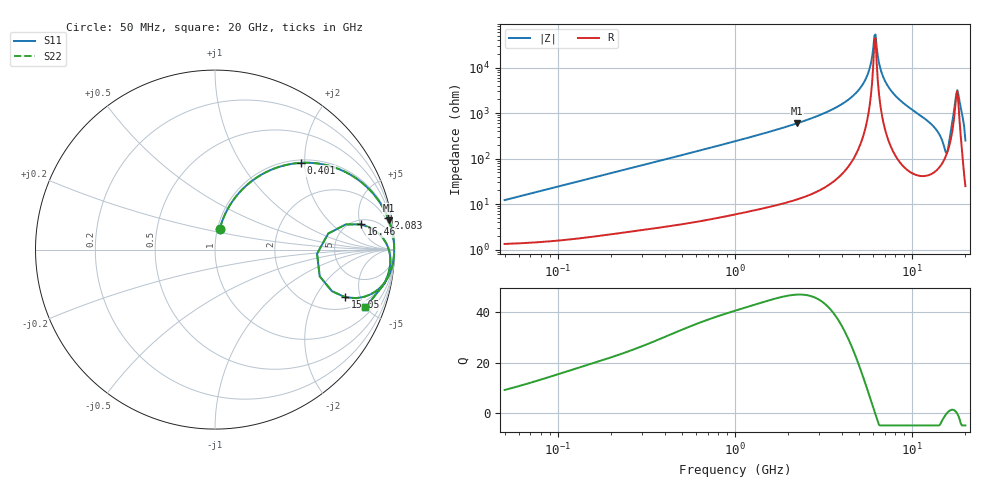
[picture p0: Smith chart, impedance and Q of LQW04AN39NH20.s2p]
!Murata Part Number: LQW04AN39NH20
!These Parameters are Measured in Series Mode Connection
!  o--[Z]--o
!Port1  Port2
!  o-------o
!Freq. Start=50[MHz] Stop=20[GHz], 401[Steps]
# Hz S RI R 50
!Freq.(Hz) S11(Real) S11(Imag) S21(Real) S21(Imag) S12(Real) S12(Imag) S22(Real) S22(Imag)
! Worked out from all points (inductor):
!   401 points, 50 MHz to 20 GHz, reference 50 ohm
!   read as one part in series: L = 38.6 nH near 51.52 MHz
!   highest Q = 47.1 at 2.245 GHz (marker M1), where L = 42.2 nH
!   self-resonance near 6.125 GHz
!   S11 on the Smith chart (normalised r, x): 50 MHz: 1.03, +0.24; 401 MHz: 1.06, +1.90; 2.083 GHz: 1, +11; 15.05 GHz: 2.76, -3.66; 16.46 GHz: 5.83, +5.15; 20 GHz: 1.49, -4.96
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5e7  0.027 0.1165  0.973 -0.1165  0.973 -0.1165  0.027 0.1165
1.364002e8  0.1101 0.287  0.8899 -0.287  0.8899 -0.287  0.1101 0.287
3.721004e8  0.4408 0.4797  0.5592 -0.4797  0.5592 -0.4797  0.4408 0.4797
4.010383e8  0.4765 0.4832  0.5235 -0.4832  0.5235 -0.4832  0.4765 0.4832
1e9  0.8458 0.3491  0.1542 -0.3491  0.1542 -0.3491  0.8458 0.3491
2.083303e9  0.9635 0.1771  0.0365 -0.1771  0.0365 -0.1771  0.9635 0.1771
2.245319e9  0.9693 0.1621  0.0307 -0.1621  0.0307 -0.1621  0.9693 0.1621
2.728004e9  0.9811 0.1259  0.0189 -0.1259  0.0189 -0.1259  0.9811 0.1259
4.966507e9  0.9974 0.0317  0.00262 -0.0317  0.00262 -0.0317  0.9974 0.0317
5.598765e9  0.9982 0.0143  0.00177 -0.0143  0.00177 -0.0143  0.9982 0.0143
6.125241e9  0.9984 0.00122  0.00158 -0.00122  0.00158 -0.00122  0.9984 0.00122
6.311513e9  0.9984 -0.00321  0.00161 0.00321  0.00161 0.00321  0.9984 -0.00321
6.802353e9  0.9981 -0.0145  0.00187 0.0145  0.00187 0.0145  0.9981 -0.0145
7.442007e9  0.9974 -0.0285  0.00261 0.0285  0.00261 0.0285  0.9974 -0.0285
1.295331e10  0.9546 -0.1702  0.0454 0.1702  0.0454 0.1702  0.9546 -0.1702
1.504638e10  0.7265 -0.2657  0.2735 0.2657  0.2735 0.2657  0.7265 -0.2657
1.573793e10  0.5686 -0.0228  0.4314 0.0228  0.4314 0.0228  0.5686 -0.0228
1.646126e10  0.8133 0.1407  0.1867 -0.1407  0.1867 -0.1407  0.8133 0.1407
1.747767e10  0.9536 0.036  0.0464 -0.036  0.0464 -0.036  0.9536 0.036
1.800918e10  0.9709 -0.00916  0.0291 0.00916  0.0291 0.00916  0.9709 -0.00916
1.855685e10  0.977 -0.0503  0.023 0.0503  0.023 0.0503  0.977 -0.0503
2e10  0.8381 -0.3219  0.1619 0.3219  0.1619 0.3219  0.8381 -0.3219
